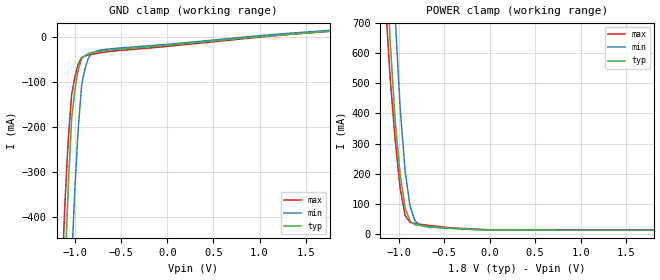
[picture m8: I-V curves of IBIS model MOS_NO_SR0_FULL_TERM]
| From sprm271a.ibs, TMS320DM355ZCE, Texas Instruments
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|   Component BCSSTL18TCSCGPBFZP33
|   Model Cell MOS_NO_SR0_FULL_TERM
[Model]   MOS_NO_SR0_FULL_TERM
Model_type   Input
Polarity   Non-Inverting
Vinl =  0.80
Vinh =  1.00
C_comp   2.680301p   2.549919p   2.900942p
[Model Spec]
Vinl   0.80   0.71   0.89
Vinh   1.00   0.91   1.09
[Temperature Range]   25   125   -40
[Voltage Range]   1.8   1.62   1.89
[POWER_clamp]
|   voltage   I(typ)   I(min)   I(max)
-1.8V     6.875A     7.433A     6.581A
-1.127V   866.7mA    1.361A     691.1mA
-1.109V   751.5mA    1.223A     603mA
-1.091V   636.4mA    1.086A     515mA
-1.036V   375.6mA    718.1mA    311.2mA
-1.018V   316.3mA    618mA      258.2mA
-981.8mV  197.8mA    418mA      152.2mA
-927.3mV  88.67mA    208.4mA    62.09mA
-872.7mV  43.33mA    92.23mA    40.11mA
-818.2mV  32.45mA    44.78mA    35.98mA
-654.5mV  26.12mA    24.15mA    29.34mA
1.8V      14.02mA    13.57mA    15.44mA
[GND_clamp]
|   voltage   I(typ)   I(min)   I(max)
-1.8V     -6.676A    -7.172A    -6.433A
-1.145V   -752.1mA   -1.249A    -557.2mA
-1.109V   -522.6mA   -980.9mA   -370.6mA
-1.073V   -332.5mA   -731.9mA   -227.6mA
-1.036V   -181.8mA   -501.8mA   -128.1mA
-1V       -115.7mA   -331.7mA   -86.98mA
-963.6mV  -70.97mA   -199.8mA   -59.29mA
-927.3mV  -47.69mA   -105.8mA   -45mA
-890.9mV  -40.68mA   -69.53mA   -41.76mA
-854.5mV  -36.09mA   -45.91mA   -39.34mA
-745.5mV  -31.59mA   -29.24mA   -35.09mA
1.764V    13.51mA    15.68mA    13.56mA
